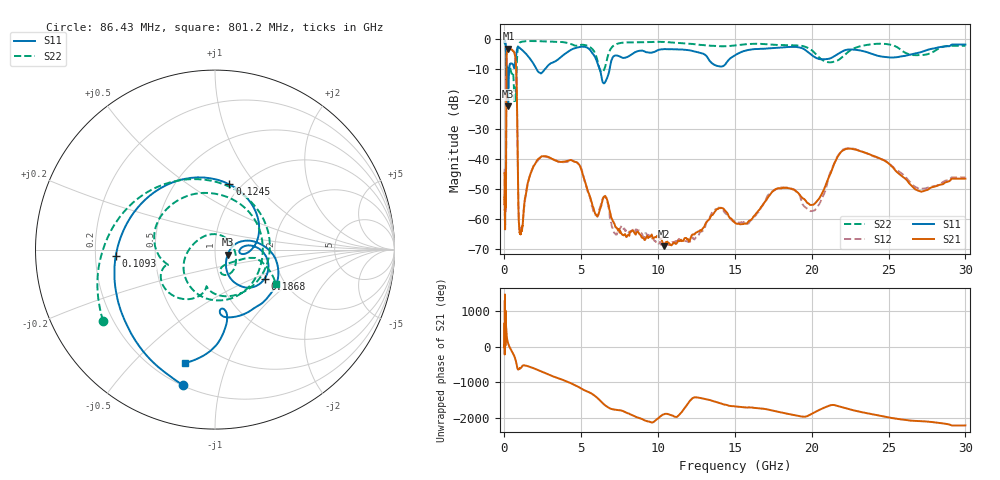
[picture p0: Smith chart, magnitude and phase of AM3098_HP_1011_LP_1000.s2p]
! Date/Time: Thu, Feb 28, 2019 8:43 AM
! Network Analyzer: Agilent Technologies E8364B Rev: A.07.50.67
! Sweep from 0.010 to 30.000 GHz, 1601 Points, Sweep Type: LOG
! Power Supply: 5.022 V, 0.002 A
# Hz S DB R 50
!freq MagS11 AngS11 MagS21 AngS21 MagS12 AngS12 MagS22 AngS22
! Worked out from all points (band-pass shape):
!   1601 points, 10 MHz to 30 GHz, reference 50 ohm
!   highest |S21| = -3.03 dB at 262.5 MHz (marker M1); lowest = -69.0 dB at 10.38 GHz (marker M2)
!   |S21| within 3 dB of the highest: 137.5 MHz to 707.1 MHz (569.6 MHz wide, 135 % of centre)
!   lowest |S11| = -22.4 dB at 242.3 MHz (marker M3), VSWR 1.16, Z = 57.5 - j3.19 ohm
!   |S11| at or under -10 dB: 190.6 MHz to 307.7 MHz (117.1 MHz wide, 47 % of centre); 2.094 GHz to 2.62 GHz (526.2 MHz wide, 22.3 % of centre); 6.207 GHz to 6.841 GHz (633.8 MHz wide, 9.72 % of centre)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
!   |S22| runs from -21.3 to -0.5 dB; largest |S21 - S12| = 0.013
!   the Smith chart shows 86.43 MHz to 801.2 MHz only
!   S11 on the Smith chart (normalised r, x): 86.43 MHz: 0.20, -0.77; 109.3 MHz: 0.29, -0.03; 124.5 MHz: 0.88, +0.74; 186.8 MHz: 1.63, -0.59; 801.2 MHz: 0.32, -0.72
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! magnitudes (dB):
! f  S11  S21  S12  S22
! 10 MHz  -0.4  -44.6  -43.1  -0.6
! 38.04 MHz  -0.4  -58.3  -59.8  -0.8
! 86.43 MHz  -2.2  -54.0  -52.6  -2.6
! 95.52 MHz  -3.2  -53.1  -56.4  -3.6
! 109.3 MHz  -5.1  -34.1  -33.9  -6.4
! 124.5 MHz  -8.6  -12.9  -12.8  -10.4
! 144.7 MHz  -17.1  -5.0  -4.9  -13.6
! 186.8 MHz  -9.9  -3.6  -3.6  -9.0
! 242.3 MHz  -22.4  -3.1  -3.0  -11.3
! 262.5 MHz  -17.0  -3.0  -3.0  -10.9
! 550.5 MHz  -8.3  -3.9  -3.8  -11.0
! 655.8 MHz  -9.3  -4.6  -4.5  -21.3
! 801.2 MHz  -3.7  -16.6  -16.5  -8.2
! 907.9 MHz  -2.5  -55.9  -55.6  -1.7
! 1.009 GHz  -2.9  -64.9  -64.8  -1.0
! 2.084 GHz  -9.9  -40.8  -41.0  -0.6
! 4.71 GHz  -2.8  -41.1  -41.1  -2.1
! 7.926 GHz  -6.0  -66.0  -64.3  -1.0
! 10.38 GHz  -3.2  -69.0  -69.1  -0.8
! 20.1 GHz  -5.6  -55.2  -57.3  -4.1
! 22.56 GHz  -3.3  -36.5  -36.4  -3.5
! 30 GHz  -1.7  -46.5  -46.1  -2.1
